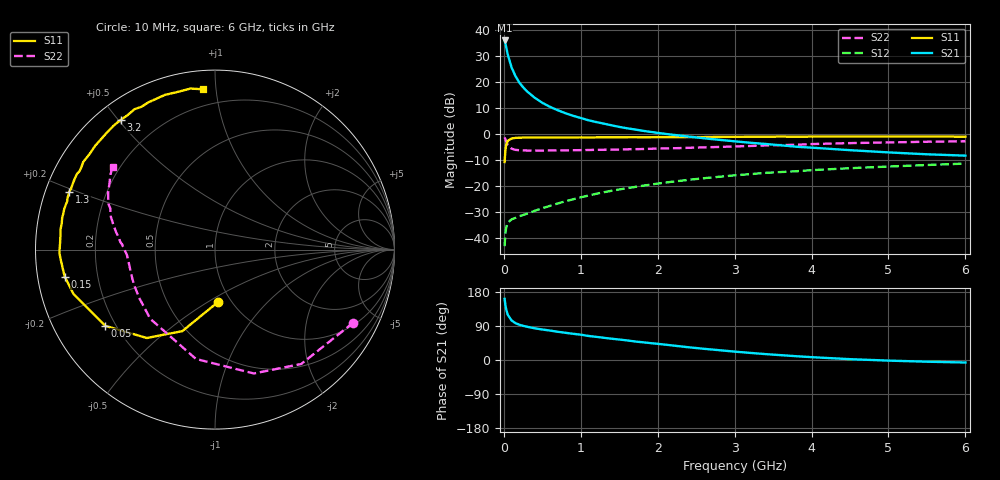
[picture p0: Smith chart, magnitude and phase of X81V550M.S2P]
! SIEMENS Small Signal Semiconductors
! BFP136W
! Si NPN RF Bipolar Junction Transistor in SOT343
! VCE = 1.5 V  IC = 50 mA
! Common Emitter S-Parameters:  September  1994
# GHz  S  MA  R  50
!  f  S11  S21  S12  S22
! GHz  MAG  ANG  MAG  ANG  MAG  ANG  MAG  ANG
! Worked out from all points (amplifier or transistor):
!   40 points, 10 MHz to 6 GHz, reference 50 ohm
!   highest |S21| = 36.1 dB at 10 MHz (marker M1)
!   |S21| within 3 dB of that: start of sweep to 33.44 MHz
!   unconditionally stable (mu >= 1): 595.9 MHz to 2.916 GHz
!   at 200 MHz: K = 0.56, MSG = 25.8 dB, |S12| = -31.6 dB
!   at 1.5 GHz: K = 1.12, MAG = 9.9 dB, |S12| = -21.3 dB
!   at 6 GHz: K = 0.98, MSG = 1.5 dB, |S12| = -11.3 dB
!   S11 on the Smith chart (normalised r, x): 10 MHz: 0.87, -0.55; 50 MHz: 0.16, -0.31; 150 MHz: 0.08, -0.09; 1.3 GHz: 0.07, +0.19; 3.2 GHz: 0.07, +0.51; 6 GHz: 0.10, +0.92
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0.01  0.2913 -86.4  63.87 161.5  0.007 70.2  0.8718 -27.8
0.02  0.4889 -111.8  55.73 145.8  0.0124 59.1  0.798 -53.0
0.03  0.6217 -127.6  47.78 134.2  0.0157 49.4  0.7232 -72.6
0.05  0.7445 -145.2  34.69 119.7  0.0197 37.3  0.6183 -99.9
0.1  0.8263 -162.6  19.41 104.4  0.023 30.4  0.528 -133.1
0.15  0.8507 -169.8  13.24 97.4  0.0245 31.5  0.5006 -147.6
0.2  0.8559 -173.6  9.951 93.3  0.0264 33.4  0.4924 -155.4
0.25  0.8623 -176.7  8.034 90.2  0.0278 37.0  0.4886 -160.3
0.3  0.8673 -178.8  6.717 87.9  0.0295 39.0  0.4858 -163.7
0.4  0.864 177.6  5.057 83.8  0.0335 43.4  0.4853 -168.1
0.5  0.8646 174.6  4.033 80.4  0.0376 47.6  0.4859 -171.0
0.6  0.8677 172.6  3.366 77.7  0.0418 50.4  0.4869 -172.8
0.7  0.8665 170.1  2.903 74.5  0.0464 52.9  0.4887 -174.2
0.9  0.8689 166.4  2.268 69.2  0.0559 55.2  0.4918 -176.6
1.1  0.8665 162.0  1.857 63.4  0.066 56.8  0.4971 -178.1
1.3  0.8738 158.3  1.599 58.6  0.0765 57.6  0.503 -179.7
1.7  0.8772 151.4  1.236 49.0  0.0964 56.6  0.5161 177.3
2.2  0.8785 143.0  0.974 38.2  0.1223 54.0  0.5369 173.6
3.2  0.8935 126.0  0.686 18.8  0.1705 45.4  0.5939 164.5
4.5  0.9061 107.9  0.493 2.2  0.222 33.3  0.6751 151.9
5.5  0.9077 98.7  0.411 -4.5  0.2556 25.3  0.7173 144.3
6  0.8957 94.3  0.387 -6.6  0.2723 20.9  0.7328 141.1
